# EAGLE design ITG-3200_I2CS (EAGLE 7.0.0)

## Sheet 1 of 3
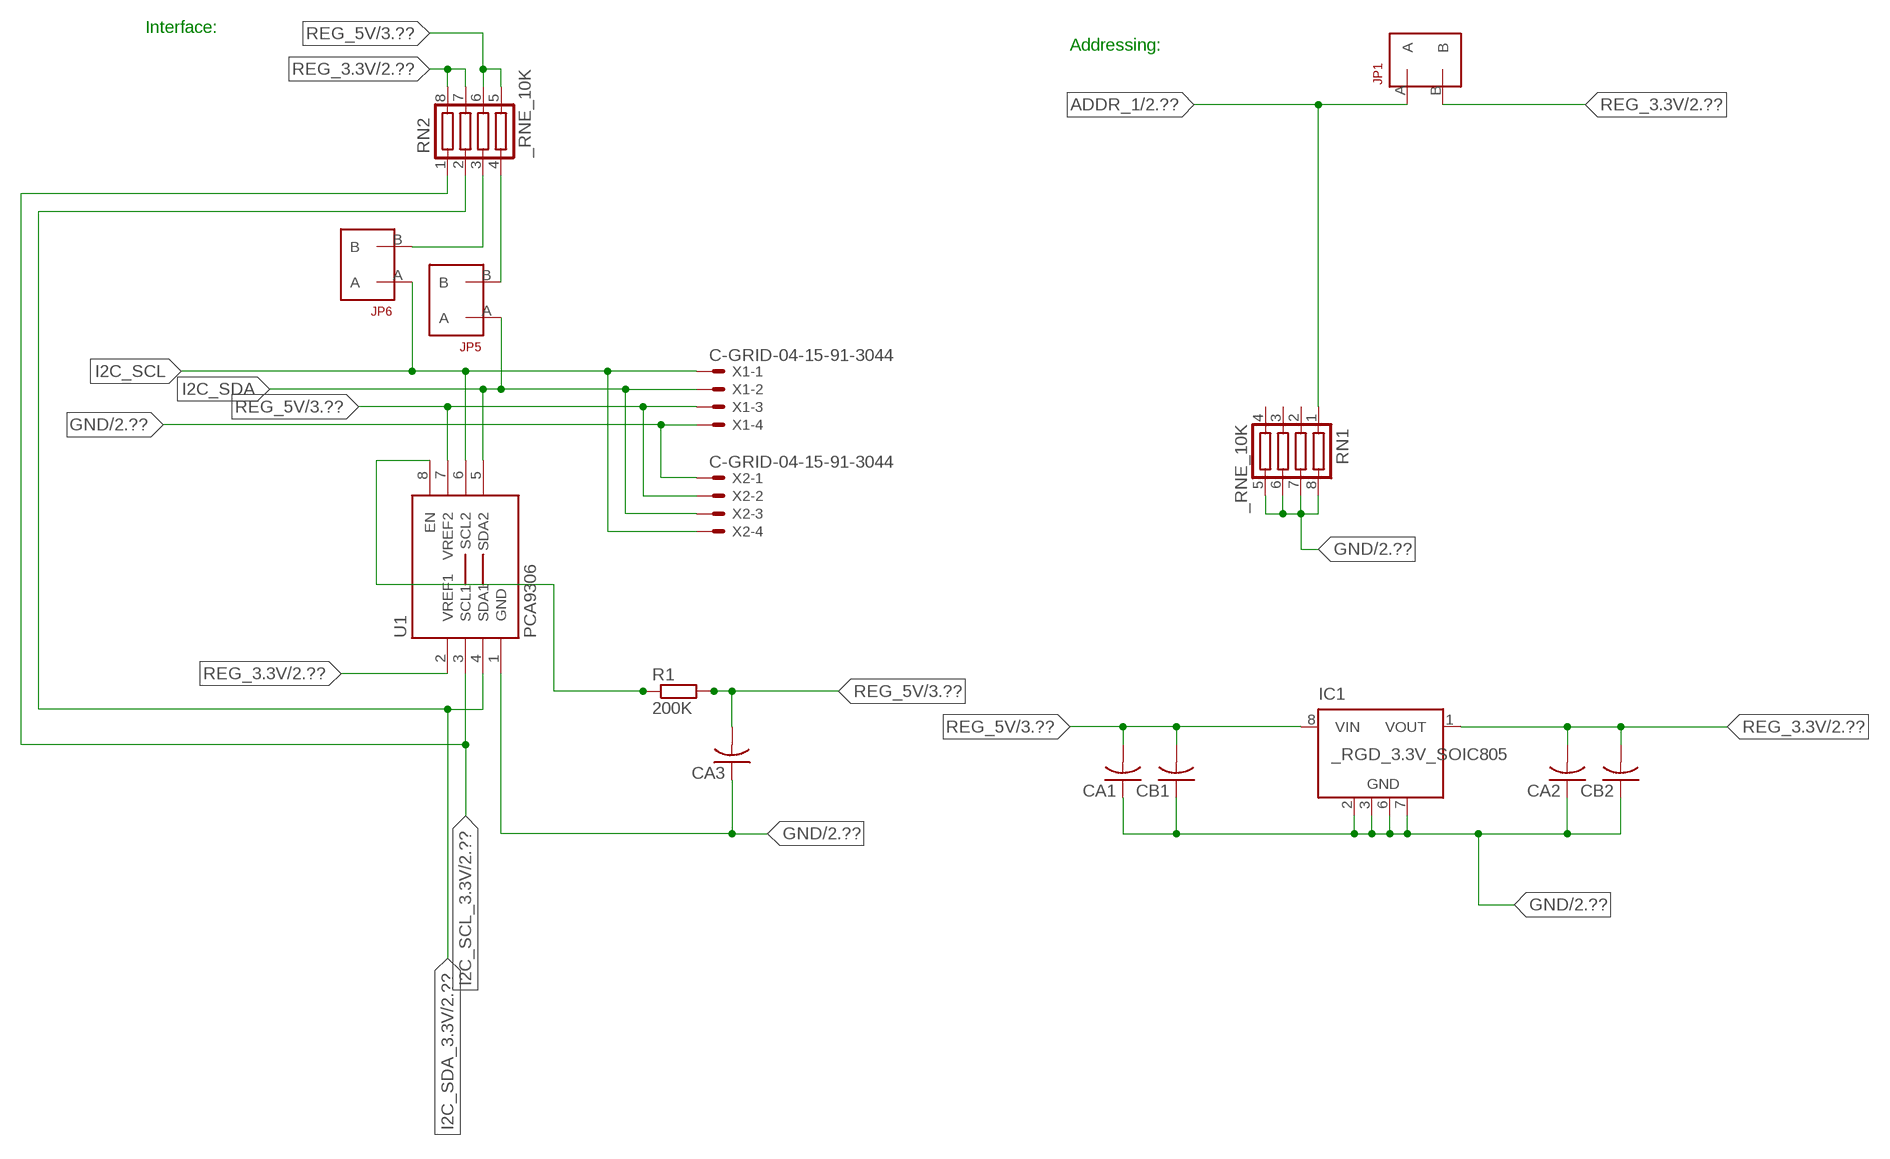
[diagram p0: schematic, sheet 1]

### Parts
CA1  CC1206KRX7R9BB104  [.1UF]
CA2  CC1206KRX7R9BB104  [.1UF]
CA3  CC1206KRX7R9BB104  [.1UF]
CB1  TMK316F106ZL-TC1206K  [TMK316F106ZL-T]
CB2  TMK316F106ZL-TC1206K  [TMK316F106ZL-T]
IC1  _RGD_3.3V_SOIC805  [_RGC_3.3V_SOIC8]
JP1  JUMPER_1X2_2MM  [JUMPER_1X2_2MM]
JP5  JUMPER_1X2_2MM  [JUMPER_1X2_2MM]
JP6  JUMPER_1X2_2MM  [JUMPER_1X2_2MM]
R1  200K  RESISTOR_SMT-0603  [R603]
RN1  _RNE_10K  [RNE]
RN2  _RNE_10K  [RNE]
U1  PCA9306  PCA9306_NCD  [PSOP-8]
X1  C-GRID-04-15-91-3044  [15-91-04]
X2  C-GRID-04-15-91-3044  [15-91-04]

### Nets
ADDR_1: JP1.A RN1.1 ; also sheet 2
GND: CA1.1 CA2.1 CA3.1 CB1.1 CB2.1 IC1.2(GND) IC1.3(GND) IC1.6(GND) IC1.7(GND) RN1.5 RN1.6 RN1.7 RN1.8 U1.1(GND) X1.4 X2.1 ; also sheet 2,3
I2C_SCL: JP6.A U1.6(SCL2) X1.1 X2.4
I2C_SCL_3.3V: RN2.1 U1.3(SCL1) ; also sheet 2
I2C_SDA: JP5.A U1.5(SDA2) X1.2 X2.3
I2C_SDA_3.3V: RN2.2 U1.4(SDA1) ; also sheet 2
N$1: JP6.B RN2.3
N$2: JP5.B RN2.4
N$3: R1.1 U1.8(EN)
REG_3.3V: CA2.2 CB2.2 IC1.1(VOUT) JP1.B RN2.7 RN2.8 U1.2(VREF1) ; also sheet 2
REG_5V: CA1.2 CA3.2 CB1.2 IC1.8(VIN) R1.2 RN2.5 RN2.6 U1.7(VREF2) X1.3 X2.2 ; also sheet 3
Unconnected: IC1.4(NC) IC1.5(NC) RN1.2 RN1.3 RN1.4

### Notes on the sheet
- Interface:
- Addressing:

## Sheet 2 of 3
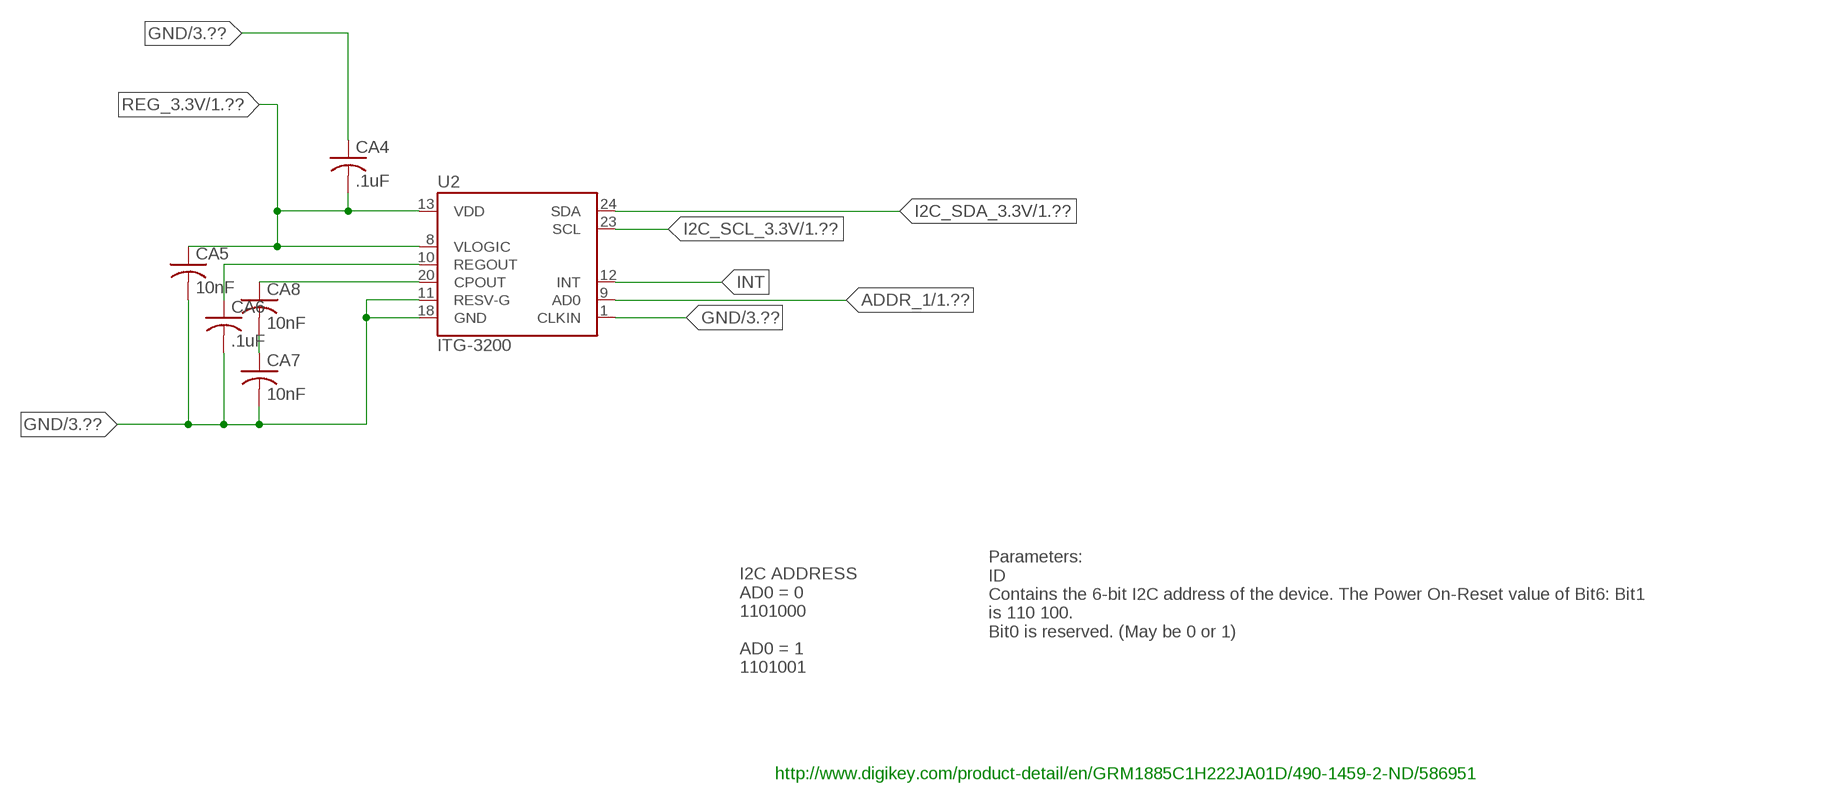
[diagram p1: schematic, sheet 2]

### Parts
CA4  .1uF  CC1206KRX7R9BB104C1206K  [CC1206KRX7R9BB104]
CA5  10nF  CC1206KRX7R9BB104C1206K  [CC1206KRX7R9BB104]
CA6  .1uF  CC1206KRX7R9BB104C1206K  [CC1206KRX7R9BB104]
CA7  10nF  _CD_10NF_50VC1206K  [_CD_10NF_50V]
CA8  10nF  _CD_10NF_50VC1206K  [_CD_10NF_50V]
U2  ITG-3200  [QFN-24]

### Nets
ADDR_1: U2.9(AD0) ; also sheet 1
GND: CA4.1 CA5.2 CA6.2 CA7.2 U2.1(CLKIN) U2.11(RESV-G) U2.18(GND) ; also sheet 1,3
I2C_SCL_3.3V: U2.23(SCL) ; also sheet 1
I2C_SDA_3.3V: U2.24(SDA) ; also sheet 1
INT: U2.12(INT)
N$4: CA7.1 CA8.2
N$6: CA6.1 U2.10(REGOUT)
N$7: CA8.1 U2.20(CPOUT)
REG_3.3V: CA4.2 CA5.1 U2.8(VLOGIC) U2.13(VDD) ; also sheet 1

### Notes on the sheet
- Parameters:
  ID
  Contains the 6-bit I2C address of the device. The Power On-Reset value of Bit6: Bit1 
  is 110 100.
  Bit0 is reserved. (May be 0 or 1)
- I2C ADDRESS
  AD0 = 0
  1101000
  
  AD0 = 1
  1101001
- http://www.digikey.com/product-detail/en/GRM1885C1H222JA01D/490-1459-2-ND/586951

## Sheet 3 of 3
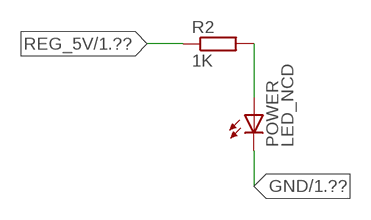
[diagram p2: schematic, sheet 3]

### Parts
POWER  LED_NCD  [CHIPLED_0603]
R2  1K  RESISTOR_SMT-0402  [R402]

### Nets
GND: POWER.C ; also sheet 1,2
N$5: POWER.A R2.2
REG_5V: R2.1 ; also sheet 1

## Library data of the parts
CA1-CA6 = NCD_ULTIMATE_LIBRARY:CC1206KRX7R9BB104: Capacitor CA .1uF 50V SMT C1206K CC1206KRX7R9BB104
CA7 CA8 = NCD_ULTIMATE_LIBRARY:_CD_10NF_50V: Capacitor 10nF SMT
CB1 CB2 = NCD_ULTIMATE_LIBRARY:TMK316F106ZL-T: Capacitor CB 10uF SMT 1206 TMK316F106ZL-T
IC1 = NCD_ULTIMATE_LIBRARY:_RGD_3.3V_SOIC8: Regulator Linear 3.3V Chip Positive VOLTAGE REGULATOR Digikey 497-1199-2-ND/L78L33ACD13TR
JP1 JP5 JP6 = NCD_ULTIMATE_CONNECTORS:JUMPER_1X2_2MM
POWER = NCD_ULTIMATE_LIBRARY:LED_NCD: LED Digikey 754-1132-2-ND/APT2012SRCPRV
R1 R2 = NCD_ULTIMATE_LIBRARY:RESISTOR_SMT: NCD Resistor
RN1 RN2 = NCD_ULTIMATE_LIBRARY:_RNE_10K: Resistor Array RNE SMT 10K x 4 Single Resistor Source: http://www.ctscorp.com/components/Datasheets/CTSChipArrayDs.pdf Digikey 742C083103JPTR-ND/742C083103JP; OC_FARNELL: unknown; OC_NEWARK: unknown
U1 = NCD_ULTIMATE_LIBRARY:PCA9306_NCD: NCD Bidirectional I2C level shifter. NOT compatible with all available part number pinout schemes- DOUBLE CHECK!!!; PROD_ID: IC-10023
U2 = NCD_ULTIMATE_bhaskar:ITG-3200: ITG-3200 3-axis gyro, digital output, qfn24 package http://store.invensense.com/ProductDetail/ITG3200-InvenSense-Inc/405256&pid=1135
X1 X2 = NCD_ULTIMATE_CONNECTORS:C-GRID-04: CONNECTOR 4-Pos I2C wire to board 2.54 mm (0.100") pitch header Digikey WM1342-ND/0015912045; OC_FARNELL: unknown; OC_NEWARK: unknown

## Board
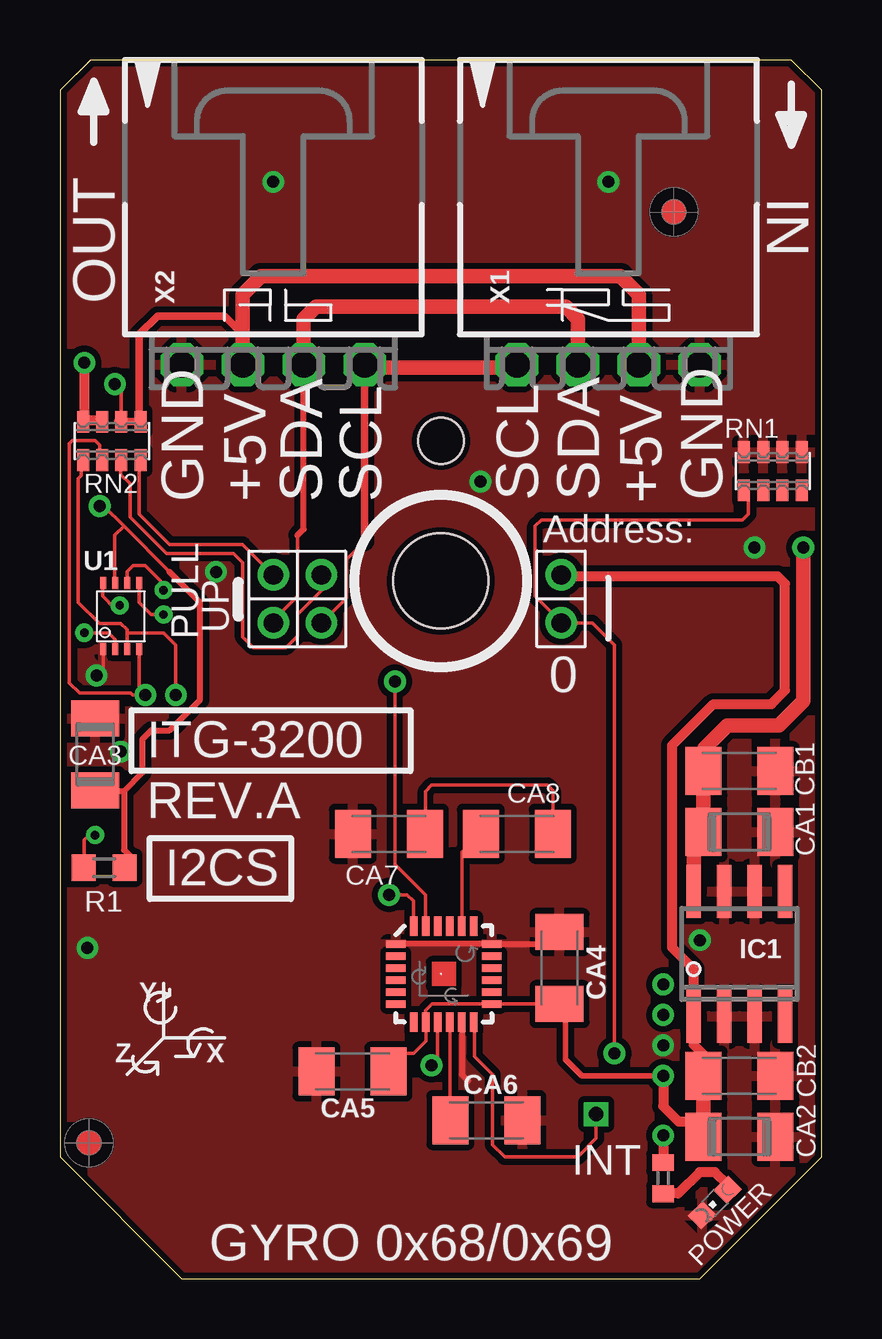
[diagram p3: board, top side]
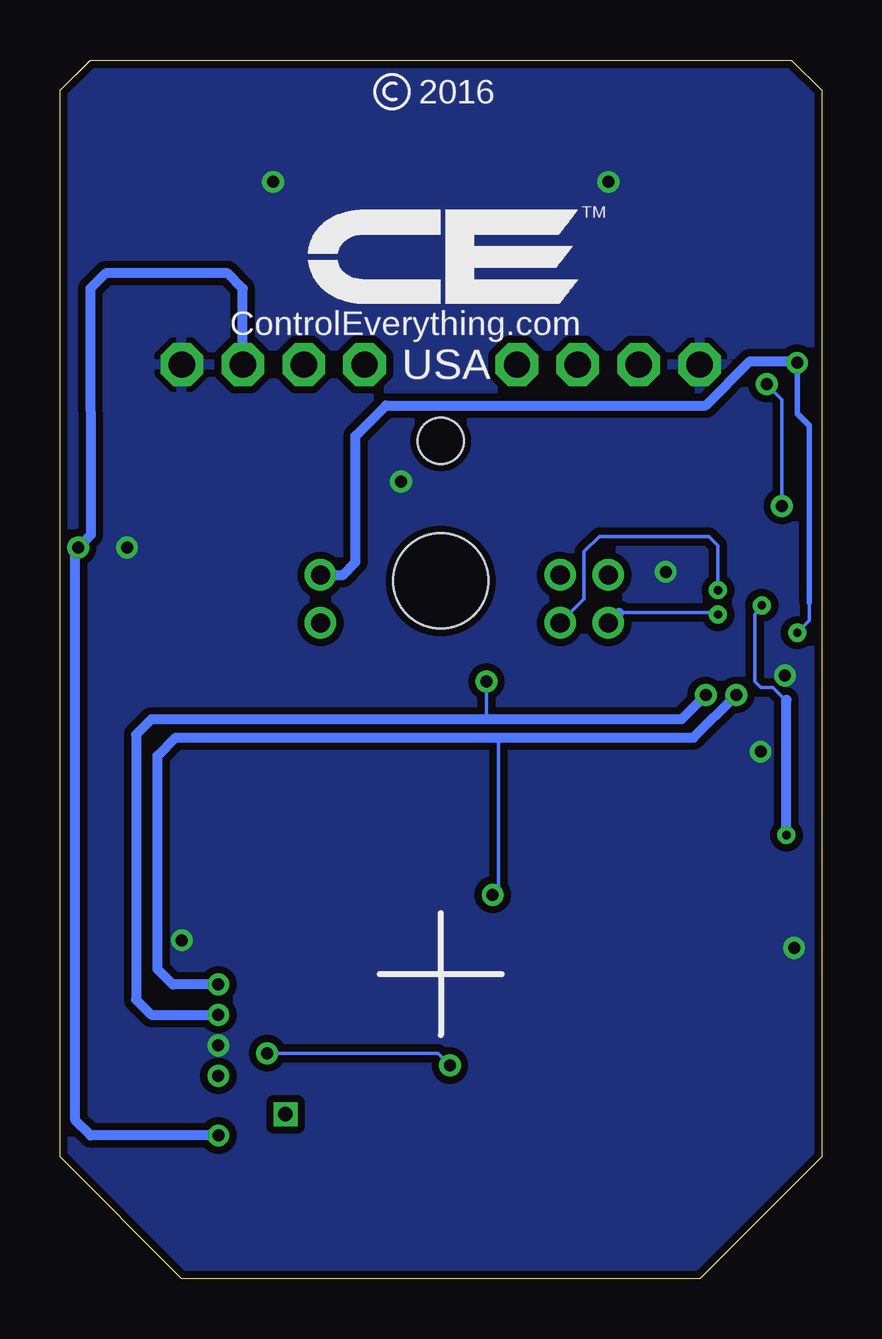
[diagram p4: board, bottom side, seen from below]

Size 31.75 x 50.8 mm. Coordinates in mm from the lower left corner, seen from the top.
Outline: 48 segments
Copper layers (1*16): Top 0.035mm / dielectric 1.5mm / Bottom 0.035mm
Design rules "default": minimum track width 5mil, minimum drill 24mil, track to track 5mil, track to pad 5mil, pad to pad 5mil, via to via 5mil, smd to smd 5mil, copper to edge 10mil, drill to drill 8mil, minimum pad ring 10mil, minimum via ring 8mil, stop-mask expansion 2mil, vias tented up to drill 0mil, thermal gap 10mil
Holes 3.96 mm at 15.88,29.08
Holes 1.91 mm at 15.88,34.93

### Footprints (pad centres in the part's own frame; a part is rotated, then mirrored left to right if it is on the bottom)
.1UF = smd 1.5 x 2: 1 -1.5,0; 2 1.5,0
CC1206KRX7R9BB104 = smd 1.5 x 2: 1 -1.5,0; 2 1.5,0
_CD_10NF_50V = smd 1.5 x 2: 1 -1.5,0; 2 1.5,0
TMK316F106ZL-T = smd 1.5 x 2: 1 -1.5,0; 2 1.5,0
_RGC_3.3V_SOIC8 = smd 0.6 x 2.2: 1 -1.905,-2.6; 2 -0.635,-2.6; 3 0.635,-2.6; 4 1.905,-2.6; 5 1.905,2.6; 6 0.635,2.6; 7 -0.635,2.6; 8 -1.905,2.6
JUMPER_1X2_2MM = drill 0.8: A 0,2; B 0,0
CHIPLED_0603 = smd 0.8 x 0.876: A 0,-0.75; C 0,0.75
R603 = smd 1 x 1.1: 1 -0.85,0; 2 0.85,0
R402 = smd 0.7 x 0.9: 1 -0.65,0; 2 0.65,0
RNE = smd 0.5 x 0.9: 1 -1.2,-0.8; 2 -0.4,-0.8; 3 0.4,-0.8; 4 1.2,-0.8; 5 1.2,0.8; 6 0.4,0.8; 7 -0.4,0.8; 8 -1.2,0.8
PSOP-8 = smd 0.25 x 0.5: 1 -0.73,-1.37; 2 -0.23,-1.37; 3 0.27,-1.37; 4 0.77,-1.37; 5 0.77,1.38; 6 0.27,1.38; 7 -0.23,1.38; 8 -0.73,1.38
QFN-24 = smd 0.8 x 0.3: 1 -2,1.25; 2 -2,0.75; 3 -2,0.25; 4 -2,-0.25; 5 -2,-0.75; 6 -2,-1.25; 13 2,-1.25; 14 2,-0.75; 15 2,-0.25; 16 2,0.25; 17 2,0.75; 18 2,1.25 | smd 0.3 x 0.8: 7 -1.25,-2; 8 -0.75,-2; 9 -0.25,-2; 10 0.25,-2; 11 0.75,-2; 12 1.25,-2; 19 1.25,2; 20 0.75,2; 21 0.25,2; 22 -0.25,2; 23 -0.75,2; 24 -1.25,2
15-91-04 = drill 1.1 pad 1.778 octagon: 1 -3.81,-7.62; 2 -1.27,-7.62; 3 1.27,-7.62; 4 3.81,-7.62

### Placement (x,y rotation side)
CA1  28.32,18.62 180 top
CA2  28.32,5.92 180 top
CA3  1.46,21.86 270 top
CA4  20.83,12.95 270 top
CA5  12.19,8.64 180 top
CA6  17.78,6.6 0 top
CA7  13.72,18.54 180 top
CA8  19.05,18.54 0 top
CB1  28.32,21.16 180 top
CB2  28.32,8.46 180 top
IC1  28.32,13.54 0 top
JP1  20.89,29.34 180 top
JP5  8.89,29.34 180 top
JP6  10.9,29.34 180 top
POWER  27.3,3.18 135 top
R1  1.84,17.13 0 top
R2  25.15,4.19 270 top
RN1  29.72,33.66 0 top
RN2  2.16,34.93 0 top
U1  2.54,27.61 0 top
U2  16,12.7 0 top
U$5  [VISION_REF10]  1.21,5.66 90 top
U$28  [VISION_REF10]  25.59,44.46 90 top
X1  22.86,45.72 0 top
X2  8.89,45.72 0 top

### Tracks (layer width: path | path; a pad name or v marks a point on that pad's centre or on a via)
ADDR_1  (via drill 0.5)
  Top 0.152: RN1.1 28.7,32.78 28.7,31.88 28.45,31.62 20.07,31.62 19.81,31.37 19.81,28.45 20.89,27.37 JP1.A 22.19,27.34 23.11,26.42 v23.11,9.4 | U2.9 15.75,9.14 v15.49,8.89
  Bottom 0.152: v15.49,8.89 16,9.4 v23.11,9.4
GND  (via drill 0.5)
  Top 0.152: CA3.1 1.52,23.42 1.52,23.62 | v1.52,25.15 1.81,25.43 U1.1
  Top 0.254: U2.1 U2.18 20.32,13.95 CA4.1 | U2.11 16.75,8.52 17.02,8.26
  other vias: 8.89,45.72 22.86,45.72 25.15,9.73 17.53,33.22 26.67,14.11 1.15,13.79 6.5,29.46 28.96,30.48 2.54,21.97
  pour Bottom (isolate 0.305): -0.64,5.08 -0.64,49.53 1.27,51.44 30.48,51.44 32.38,49.53 32.38,5.08 26.67,-0.63 5.08,-0.63
  pour Top (isolate 0.254): 4.45,-1.27 -1.27,4.45 -1.27,50.17 0.64,52.07 31.11,52.07 33.02,50.17 33.02,4.45 27.3,-1.27
I2C_SCL  (via drill 0.35)
  Top 0.152: 12.7,30.73 11.94,29.97 11.94,28.38 JP6.A | v4.32,28.7 4.32,28.96 3.56,29.72 3.05,29.72 2.81,29.48 U1.6
  Top 0.305: 12.7,30.73 X2.4
  Top 0.406: X2.4 12.7,37.97 | 19.05,37.97 X1.1
  Top 0.61: 12.7,37.97 19.05,37.97
  Bottom 0.152: JP6.A 9.91,28.33 9.91,30.3 9.27,30.94 4.7,30.94 4.32,30.55 v4.32,28.7
I2C_SCL_3.3V  (via drill 0.5)
  Top 0.152: RN2.1 0.89,34.07 0.89,33.48 0.77,33.35 0.77,28.19 1.65,27.31 2.54,27.31 2.79,27.05 2.79,26.92 | U2.23 15.24,14.71 15.24,16 13.97,17.27 v13.97,24.89 | 2.79,26.92 2.81,26.91 U1.3 2.79,26.25 2.79,26.92 | 2.79,26.92 4.32,26.92 4.83,26.41 v4.83,24.33
  Bottom 0.152: v13.97,24.89 13.97,23.32
  Bottom 0.406: v4.83,24.33 5.84,23.32 13.97,23.32 27.94,23.32 28.58,22.68 28.58,11.63 27.94,11 v25.15,11
I2C_SDA  (via drill 0.35)
  Top 0.152: JP5.A 8.89,27.44 9.91,28.45 9.91,30.99 | U1.5 3.3,28.19 3.81,27.69 v4.32,27.69
  Top 0.254: 9.91,30.99 10.16,31.25 X2.3
  Top 0.61: X2.3 10.16,40.01 10.67,40.51 21.09,40.51 21.59,40.01 X1.2
  Bottom 0.152: v4.32,27.69 4.39,27.76 8.44,27.76
  Bottom 0.406: 8.44,27.76 JP5.A
I2C_SDA_3.3V  (via drill 0.5)
  Top 0.152: RN2.2 1.65,34.14 1.65,34.75 1.46,34.94 0.51,34.94 0.38,34.81 0.38,26.54 0.38,24.84 0.81,24.41 2.95,24.41 3.02,24.33 v3.56,24.33 3.35,24.33 3.31,24.38 U1.4 3.3,25.4 | U2.24 14.73,14.72 14.73,15.75 14.48,16 v13.72,16
  Bottom 0.152: v13.72,16 13.46,16.26 13.46,22.56
  Bottom 0.406: v25.15,12.27 27.05,12.27 27.69,12.9 27.69,21.79 26.93,22.56 13.46,22.56 5.34,22.56 v3.56,24.33
INT  (via drill 0.6)
  Top 0.152: U2.12 17.27,10.68 17.27,9.27 18.03,8.51 18.03,5.59 18.54,5.08 21.59,5.08 22.35,5.84 v22.35,6.86
N$1
  Top 0.152: JP6.B 10.92,29.31 10.92,28.7 9.91,27.69 9.91,26.8 9.42,26.31 8.06,26.31 7.62,26.75 7.62,29.84 7.24,30.23 4.45,30.23 2.92,31.75 2.92,33.15 2.54,33.53 2.54,34.1 RN2.3
  Top 0.305: 2.54,34.02 RN2.3
N$2
  Top 0.152: JP5.B 7.62,30.61 4.57,30.61 3.3,31.88 3.3,34.07 RN2.4
  Top 0.305: 3.37,33.88 RN2.4
N$3  (via drill 0.35)
  Top 0.152: 1.02,17.16 1.02,18.29 1.46,18.74 v1.46,18.49 | U1.8 1.78,28.96 1.78,28.45 2.29,27.94 v2.49,28.07
  Top 0.406: R1.1 1.02,17.13 1.02,17.16
  Bottom 0.152: v2.49,28.07 2.79,27.69 2.79,24.89 2.54,24.64 2.03,24.64 1.54,24.14 1.46,24.14
  Bottom 0.406: v1.46,18.49 1.46,24.14
N$4
  Top 0.152: CA7.1 15.24,18.57 15.24,20.32 15.49,20.57 20.32,20.57 20.55,20.34 CA8.2
N$5
  Top 0.406: POWER.A 27.84,3.92 27.3,4.45 26.67,4.45 25.78,3.56 25.16,3.56 R2.2
N$6
  Top 0.152: U2.10 16.26,7.37 16.28,7.34 CA6.1
N$7
  Top 0.152: U2.20 16.76,14.71 16.76,17.78 17.04,18.06 CA8.1
REG_3.3V  (via drill 0.35, 0.5)
  Top 0.152: 21.08,11.2 CA4.2 U2.13 15.51,11.45 15.24,11.18 15.24,10.71 U2.8 15.25,9.92 14.73,9.4 14.45,9.4 CA5.1 | v1.02,26.92 2.03,26.92 2.31,26.65 U1.2
  Top 0.229: 21.08,11.2 21.08,9.14 21.77,8.46 v25.15,8.46
  Top 0.406: CB2.2 26.82,9.35 26.42,9.75 26.42,10.36 | v25.15,8.46 25.15,7.19 25.78,6.55 26.82,6.55 | IC1.1 26.42,12.9 25.53,13.79 25.53,22.24 27.24,23.95 29.66,23.95 30.23,24.52 30.23,28.97 29.91,29.29 20.95,29.29 JP1.B | 26.52,5.62 CA2.2 | v1.02,38.18 1.02,35.78 | 1.02,35.78 RN2.8 | 1.02,35.78 1.71,35.78 RN2.7
  Top 0.61: CB2.2 26.82,6.55 CA2.2 | 26.42,10.36 IC1.1
  Bottom 0.152: 0.51,28.19 0.51,27.43 v1.02,26.92
  Bottom 0.229: 0.51,28.19 0.51,35.56 1.02,36.07 v1.02,38.18
  Bottom 0.406: v1.02,38.18 1.08,38.24 2.99,38.24 4.83,36.4 18.16,36.4 19.43,35.13 19.43,29.87 19.94,29.34 JP1.B
REG_5V  (via drill 0.5)
  Top 0.152: RN2.6 2.56,37.01 v2.29,37.29 | R1.2 3.05,17.49 | 4.57,29.46 2.67,31.37 | 2.67,31.37 1.83,32.21 v1.65,32.21 | U1.7 2.29,29.01 2.29,30.99 2.67,31.37
  Top 0.254: 2.67,20.32 3.43,21.08 3.43,22.48 3.81,22.86 4.57,22.86 5.84,24.13 5.84,28.19 4.57,29.46 | 2.67,20.32 1.5,20.32 CA3.2 | 2.67,20.32 2.67,17.87 3.05,17.49
  Top 0.305: 7.62,39.37 7.5,39.37 | 2.42,35.74 RN2.6 RN2.5 3.31,35.8 3.31,39.37 4.07,40.13 6.86,40.13 7.62,39.37 | X2.2 7.62,39.37
  Top 0.406: v25.15,5.97 R2.1
  Top 0.61: X2.2 7.62,41.02 8.38,41.78 23.37,41.78 24.13,41.02 X1.3 | IC1.8 26.42,18.21 CA1.2 CB1.2 26.86,21.2 26.86,22.11 27.82,23.06 29.98,23.06 30.99,24.08 v30.99,30.48
  Bottom 0.152: v1.65,32.21 1.65,36.65 v2.29,37.29
  Bottom 0.406: X1.3 24.13,41.28 24.77,41.91 29.84,41.91 30.48,41.27 30.47,31 v30.99,30.48 31.11,30.36 31.11,6.6 30.48,5.97 v25.15,5.97

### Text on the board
tPlace: Y | Z | X
tNames: IN | OUT | GND | +5V | SDA | SCL | SCL | SDA | +5V | GND | Address: | PULL | UP | 0 | ITG-3200 | REV.A | I2CS | INT | GYRO 0x68/0x69
bNames: 2016 | TM | ControlEverything.com | USA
